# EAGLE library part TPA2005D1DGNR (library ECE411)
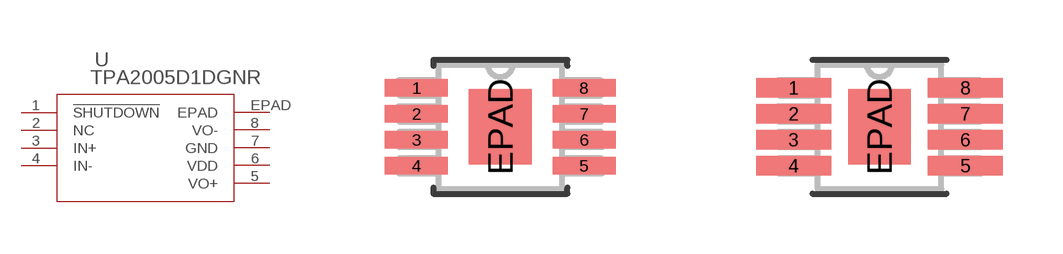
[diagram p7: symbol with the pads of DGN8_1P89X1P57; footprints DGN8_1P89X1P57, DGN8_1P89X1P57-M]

Designator prefix U

## TPA2005D1DGNR (MANUFACTURER_PART_NUMBER: TPA2005D1DGNR; VENDOR: Texas Instruments)  [DGN8_1P89X1P57]
1  !SHUTDOWN  in
2  NC  pas
3  IN+  in
4  IN-  in
5  VO+  out
6  VDD  pwr
7  GND  pwr
8  VO-  out
EPAD  EPAD  pas

## TPA2005D1DGNRDGN8_1P89X1P57-M (MANUFACTURER_PART_NUMBER: TPA2005D1DGNR; VENDOR: Texas Instruments)  [DGN8_1P89X1P57-M]
Pads as for DGN8_1P89X1P57

## TPA2005D1DGNRDGN8_1P89X1P57-L (MANUFACTURER_PART_NUMBER: TPA2005D1DGNR; VENDOR: Texas Instruments)  [DGN8_1P89X1P57-L]
Pads as for DGN8_1P89X1P57

## Footprint DGN8_1P89X1P57 (pad centres in mm)
smd 1.575 x 0.432: 1 -2.095,0.975; 2 -2.095,0.325; 3 -2.095,-0.325; 4 -2.095,-0.975; 5 2.095,-0.975; 6 2.095,-0.325; 7 2.095,0.325; 8 2.095,0.975
smd 1.57 x 1.89: EPAD 0,0

## Footprint DGN8_1P89X1P57-M (pad centres in mm)
smd 1.88 x 0.483: 1 -2.146,0.975; 2 -2.146,0.325; 3 -2.146,-0.325; 4 -2.146,-0.975; 5 2.146,-0.975; 6 2.146,-0.325; 7 2.146,0.325; 8 2.146,0.975
smd 1.57 x 1.89: EPAD 0,0

## Footprint DGN8_1P89X1P57-L (pad centres in mm)
smd 1.27 x 0.381: 1 -2.045,0.975; 2 -2.045,0.325; 3 -2.045,-0.325; 4 -2.045,-0.975; 5 2.045,-0.975; 6 2.045,-0.325; 7 2.045,0.325; 8 2.045,0.975
smd 1.57 x 1.89: EPAD 0,0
